PROGRAM MAIN
VAR
	Axis_A: axis_ref;
	Axis_B: axis_ref;
	
	axis_a_Dctime AT %I*:t_dctime32;
	Di AT %I*:INT;
	SignalTrig:Tc2_Standard.R_TRIG;
	
	
	MC_TouchProbe1: MC_TouchProbe;//A轴 touchprobe
	MC_TouchProbe2: MC_TouchProbe;//B轴 touchprobe
	MC_AbortTrigger1: MC_AbortTrigger;
	
	XFCPositionAtTime1:XFC_PositionAtTime;
	ConvertDcTimeToPos1:ConvertDcTimeToPos;

	TriggerInput	: TRIGGER_REF; 		(* Reference to the trigger signal source. *)
	TriggerInput2: TRIGGER_REF;
	
	bAbort: BOOL;

	bLatch: BOOL;
	MC_Power1: MC_Power;
	MC_MoveVelocity1: MC_MoveVelocity;
	bMove: BOOL;
	ENABLE: BOOL;
	Ready: BOOL;
	MC_Stop1: MC_Stop;
	bStop: BOOL;
	MC_Reset1: MC_Reset;
	bReset: BOOL;
	SoEReset1: FB_SoEReset;

	Trigactpos: LREAL; //上升沿获取到的位置
	Axis_A_TouchRecordedPos: LREAL;
	Axis_B_TouchRecordedPos: LREAL;//touchprobe获取到的B轴位置

	Axis_B_DctimePos: LREAL;
	Axis_B_XFCDctimePos: LREAL;
	DcTimeDiff: LREAL;
	
	Touch_ActposDiff: LREAL;
	Dcpos_ActposDiff: LREAL;
	Touch_DcposDiff: LREAL;	
END_VAR

Motion();
Axis_A.ReadStatus();
TriggerInput.EncoderID:=Axis_A.NcToPlc.AxisId;
TriggerInput2.EncoderID:=Axis_B.NcToPlc.AxisId;
TouchProbe();

IF MC_TouchProbe1.Done THEN
bLatch:=FALSE;
XFCPositionAtTime1(
	DcTime:= axis_a_Dctime, 
	Options:= , 
	Position=>Axis_B_XFCDctimePos , 
	Error=> , 
	ErrorID=> , 
	Axis:=Axis_B );
ConvertDcTimeToPos1(
	nAxisId:=Axis_B.NcToPlc.AxisId , 
	nSubIdx:=0 , 
	dcTime:=axis_a_Dctime , 
	fPosition=>Axis_B_DctimePos , 
	iErr=> );

END_IF
	
SignalTrig(CLK:= Di.1 , Q=> );
IF SignalTrig.Q THEN
		Trigactpos:=Axis_B.NcToPlc.ActPos;
END_IF

DcTimeDiff:=	Axis_B_XFCDctimePos - Axis_B_DctimePos;

Touch_ActposDiff:=Axis_B_TouchRecordedPos - Trigactpos;
Dcpos_ActposDiff:=Axis_B_XFCDctimePos - Trigactpos;
Touch_DcposDiff:=Axis_B_TouchRecordedPos - Axis_B_XFCDctimePos;

ACTION motion:
MC_Power1(
	Axis:=Axis_A, 
	Enable:=1, 
	Enable_Positive:= 1, 
	Enable_Negative:=1 , 
	Override:= , 
	BufferMode:= , 
	Options:= , 
	Status=> , 
	Busy=> , 
	Active=> , 
	Error=> , 
	ErrorID=> );
	
MC_Power1(
	Axis:=Axis_B , 
	Enable:=1, 
	Enable_Positive:= 1, 
	Enable_Negative:=1 , 
	Override:= , 
	BufferMode:= , 
	Options:= , 
	Status=> , 
	Busy=> , 
	Active=> , 
	Error=> , 
	ErrorID=> );
	

MC_MoveVelocity1(
	Axis:=Axis_B  , 
	Execute:=bMove , 
	Velocity:=360*5 , 
	Acceleration:= , 
	Deceleration:= , 
	Jerk:= , 
	Direction:= , 
	BufferMode:= , 
	Options:= , 
	InVelocity=> , 
	Busy=> , 
	Active=> , 
	CommandAborted=> , 
	Error=> , 
	ErrorID=> );	
	
	
	
MC_Reset1(
	Axis:=Axis_A , 
	Execute:=bReset , 
	Done=> , 
	Busy=> , 
	Error=> , 
	ErrorID=> );
END_ACTION

ACTION TouchProbe:
MC_TouchProbe1(
	Axis:= Axis_A, 
	TriggerInput:=TriggerInput , 
	Execute:= bLatch, 
	WindowOnly:= , 
	FirstPosition:= , 
	LastPosition:= , 
	Done=> , 
	Busy=> , 
	CommandAborted=> , 
	Error=> , 
	ErrorID=> , 
	RecordedPosition=> Axis_A_TouchRecordedPos, 
	RecordedData=> );
MC_TouchProbe2(
	Axis:= Axis_B, 
	TriggerInput:=TriggerInput2 , 
	Execute:= bLatch, 
	WindowOnly:= , 
	FirstPosition:= , 
	LastPosition:= , 
	Done=> , 
	Busy=> , 
	CommandAborted=> , 
	Error=> , 
	ErrorID=> , 
	RecordedPosition=> Axis_B_TouchRecordedPos, 
	RecordedData=> );
	
	
MC_AbortTrigger1(
	Axis:=Axis_A , 
	TriggerInput:= TriggerInput, 
	Execute:= bAbort, 
	Done=> , 
	Busy=> , 
	Error=> , 
	ErrorID=> );
END_ACTION

END_PROGRAM
